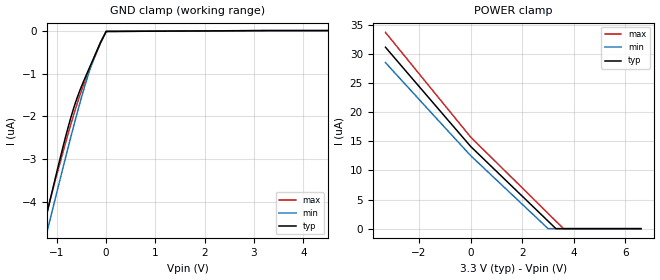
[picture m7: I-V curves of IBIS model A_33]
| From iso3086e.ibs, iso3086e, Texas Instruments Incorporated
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|   A_33 MODEL
[Model]   A_33
Model_type   Input
|Signals   A   positive pin
|Rref = 27   Note: 54 Ohm differential load;
Vinl   = 0.8
Vinh   = 2
| C_comp   obtained at 20MHz
|   typ   min   max
C_comp   5.326fF   5.258fF   5.400fF
[Voltage Range]   3.3   3   3.6
[Temperature Range]   40   125   -40
[Power Clamp Reference]   3.3   3   3.6
[GND Clamp Reference]   0   0   0
[GND Clamp]
|   Voltage   I(typ)   I(min)   I(max)
-3.3V     -14.97uA   -14.79uA   -15.11uA
-1.33V    -4.904uA   -5.312uA   -4.815uA
-1.241V   -4.463uA   -4.893uA   -4.413uA
-1.191V   -4.22uA    -4.661uA   -4.194uA
-864.6mV  -2.669uA   -3.151uA   -2.791uA
-740.9mV  -2.133uA   -2.594uA   -2.288uA
-636.9mV  -1.735uA   -2.138uA   -1.886uA
-498.3mV  -1.3uA     -1.555uA   -1.399uA
-290.4mV  -743.1nA   -784.8nA   -784.4nA
-117.2mV  -290.2nA   -282.6nA   -306.7nA
1.65mV    -20.01nA   -20.02nA   -19.91nA
6.6V      0A         0A         0A
[POWER Clamp]
|   Voltage   I(typ)   I(min)   I(max)
-3.3V     31.13uA    28.49uA    33.67uA
1.65mV    14.1uA     12.53uA    15.71uA
3.001V    1.289uA    0A         2.614uA
3.303V    0A         0A         1.296uA
3.6V      0A         0A         0A
6.6V      0A         0A         0A
